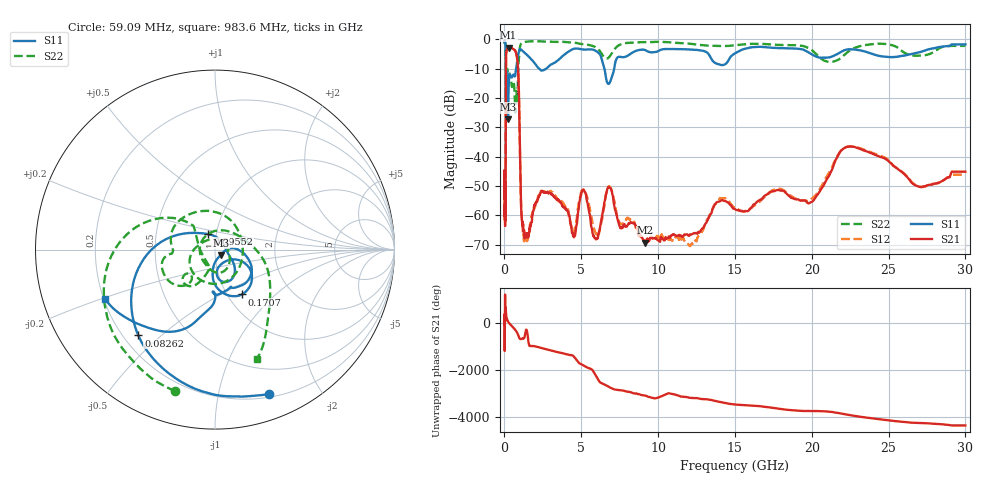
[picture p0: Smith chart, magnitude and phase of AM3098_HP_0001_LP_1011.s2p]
! Date/Time: Thu, Feb 28, 2019 8:32 AM
! Network Analyzer: Agilent Technologies E8364B Rev: A.07.50.67
! Sweep from 0.010 to 30.000 GHz, 1601 Points, Sweep Type: LOG
! Power Supply: 5.022 V, 0.002 A
# Hz S DB R 50
!freq MagS11 AngS11 MagS21 AngS21 MagS12 AngS12 MagS22 AngS22
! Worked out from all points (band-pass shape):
!   1601 points, 10 MHz to 30 GHz, reference 50 ohm
!   highest |S21| = -2.81 dB at 269.1 MHz (marker M1); lowest = -69.3 dB at 9.164 GHz (marker M2)
!   |S21| within 3 dB of the highest: 105.6 MHz to 807 MHz (701.4 MHz wide, 154 % of centre)
!   lowest |S11| = -27.2 dB at 232.8 MHz (marker M3), VSWR 1.09, Z = 53.2 - j3.12 ohm
!   |S11| at or under -10 dB: 91.07 MHz to 756.2 MHz (665.2 MHz wide, 157 % of centre); 2.273 GHz to 2.712 GHz (438.7 MHz wide, 17.6 % of centre); 6.505 GHz to 7.141 GHz (635.2 MHz wide, 9.31 % of centre)
!   |S22| runs from -24.9 to -0.6 dB; largest |S21 - S12| = 0.01
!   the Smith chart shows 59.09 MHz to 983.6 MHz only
!   S11 on the Smith chart (normalised r, x): 59.09 MHz: 0.23, -1.42; 82.62 MHz: 0.26, -0.42; 95.52 MHz: 0.91, +0.16; 170.7 MHz: 1.16, -0.64; 983.6 MHz: 0.21, -0.21
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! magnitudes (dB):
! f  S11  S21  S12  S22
! 10 MHz  -0.3  -44.7  -46.2  -0.6
! 38.04 MHz  -0.5  -59.5  -61.8  -1.0
! 59.09 MHz  -1.3  -55.5  -50.6  -1.7
! 71.1 MHz  -2.0  -54.3  -53.8  -2.5
! 82.62 MHz  -3.9  -32.9  -32.3  -4.3
! 95.52 MHz  -20.3  -10.2  -10.2  -21.9
! 144.7 MHz  -14.6  -3.5  -3.5  -12.9
! 170.7 MHz  -10.7  -3.4  -3.3  -10.1
! 232.8 MHz  -27.2  -2.9  -2.9  -12.4
! 269.1 MHz  -16.7  -2.8  -2.8  -12.6
! 550.5 MHz  -12.2  -3.2  -3.2  -14.6
! 850.8 MHz  -6.6  -7.6  -7.6  -19.1
! 983.6 MHz  -3.5  -31.1  -31.0  -3.7
! 1.093 GHz  -3.5  -58.4  -57.7  -1.4
! 1.251 GHz  -4.3  -65.7  -66.8  -0.9
! 2.084 GHz  -8.9  -55.5  -55.9  -0.6
! 6.821 GHz  -15.0  -50.6  -50.0  -6.0
! 7.926 GHz  -5.8  -63.8  -61.3  -1.2
! 9.164 GHz  -3.6  -69.3  -68.8  -0.9
! 19.7 GHz  -4.1  -55.7  -55.3  -2.7
! 22.67 GHz  -3.4  -36.6  -36.6  -3.1
! 30 GHz  -1.7  -45.1  -46.1  -2.2
